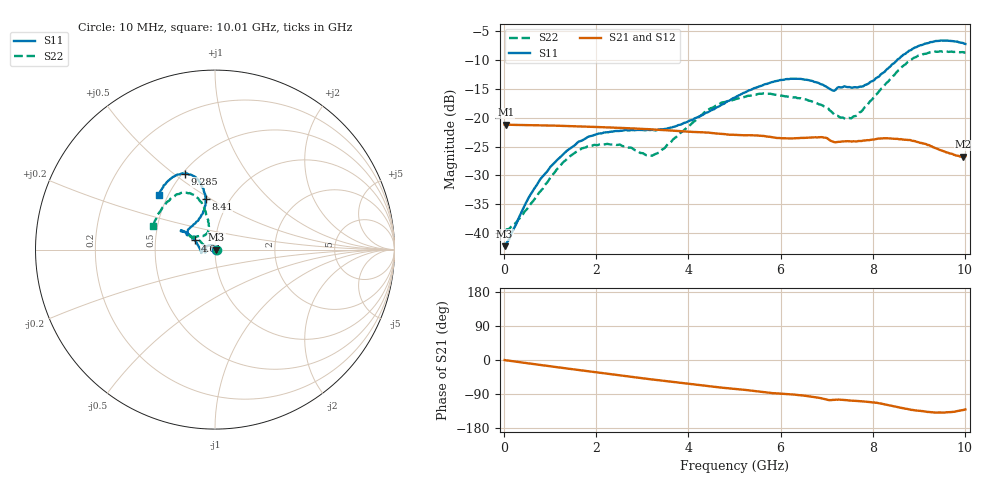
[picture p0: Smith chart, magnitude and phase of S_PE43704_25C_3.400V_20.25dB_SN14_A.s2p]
! Device ID: PE43704
! Dir: z:\PE43704\PE43704_Char_1_20130516\PE43704\AMB\3p400V\20p25dB
! Serial: 14
! Insertion: A
! Impedance: 50 ohm
! Temp: Amb
! VDD: 3.400V
! Attenuation Step: 20.25dB
! IDD: 1.139926e-01mA
#  Hz  S  RI  R  50
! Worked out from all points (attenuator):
!   401 points, 10 MHz to 10.01 GHz, reference 50 ohm
!   highest |S21| = -21.20 dB at 35 MHz (marker M1); lowest = -26.7 dB at 9.96 GHz (marker M2)
!   lowest |S11| = -42.3 dB at 10 MHz (marker M3), VSWR 1.02, Z = 50.8 + j0.0405 ohm
!   |S11| at or under -10 dB: start of sweep to 8.526 GHz
!   |S22| runs from -39.7 to -8.5 dB; largest |S21 - S12| = 0.00083
!   S11 on the Smith chart (normalised r, x): 10 MHz: 1.02, +0.00; 4.61 GHz: 0.80, +0.08; 8.41 GHz: 0.77, +0.48; 9.285 GHz: 0.52, +0.55; 10.01 GHz: 0.45, +0.33
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1e7  0.00769 0.000399  0.0871 -0.00033  0.0872 -0.00025  0.0104 0.000286
3.5e7  0.00782 0.00156  0.0871 -0.000934  0.0871 -0.000966  0.0105 0.00121
2.85e8  0.00465 0.0117  0.0864 -0.00734  0.0863 -0.00733  0.00738 0.0104
7.85e8  -0.0156 0.0249  0.0837 -0.0195  0.0837 -0.0194  -0.012 0.0196
1.285e9  -0.044 0.0199  0.0793 -0.0307  0.0792 -0.0306  -0.0393 0.0124
1.685e9  -0.063 0.00716  0.0745 -0.0389  0.0745 -0.0389  -0.0541 -0.00123
2.26e9  -0.074 -0.0114  0.0662 -0.0491  0.0662 -0.0491  -0.0571 -0.0154
3.135e9  -0.0768 -0.0158  0.0509 -0.0611  0.051 -0.061  -0.0472 -0.000939
3.36e9  -0.0786 -0.00987  0.0467 -0.0632  0.0467 -0.0632  -0.0492 0.00817
4.61e9  -0.1117 0.051  0.0231 -0.0693  0.0232 -0.0692  -0.1078 0.0691
5.01e9  -0.1313 0.0725  0.0166 -0.069  0.0168 -0.0691  -0.1263 0.0707
5.96e9  -0.1823 0.1052  0.00194 -0.0667  0.00206 -0.0666  -0.1405 0.0692
6.685e9  -0.1829 0.1004  -0.00822 -0.0668  -0.00807 -0.0669  -0.1217 0.065
7.135e9  -0.1499 0.0848  -0.0163 -0.0599  -0.0163 -0.0599  -0.0812 0.0738
7.51e9  -0.1323 0.1275  -0.0184 -0.0597  -0.0181 -0.0596  -0.0488 0.086
7.86e9  -0.0879 0.1731  -0.0218 -0.0599  -0.0216 -0.06  -0.0352 0.1208
8.36e9  -0.0522 0.2689  -0.0329 -0.0574  -0.0328 -0.0575  -0.0504 0.2059
8.41e9  -0.0529 0.2825  -0.0337 -0.0565  -0.0339 -0.0568  -0.0569 0.2168
8.86e9  -0.0911 0.3845  -0.042 -0.0471  -0.0413 -0.0473  -0.1156 0.3031
9.285e9  -0.1661 0.4218  -0.0419 -0.0378  -0.0422 -0.0376  -0.1984 0.3103
9.96e9  -0.3058 0.3228  -0.0309 -0.0342  -0.0312 -0.0339  -0.3388 0.1511
1.001e10  -0.3132 0.3041  -0.0301 -0.0353  -0.0307 -0.0355  -0.3443 0.1309
